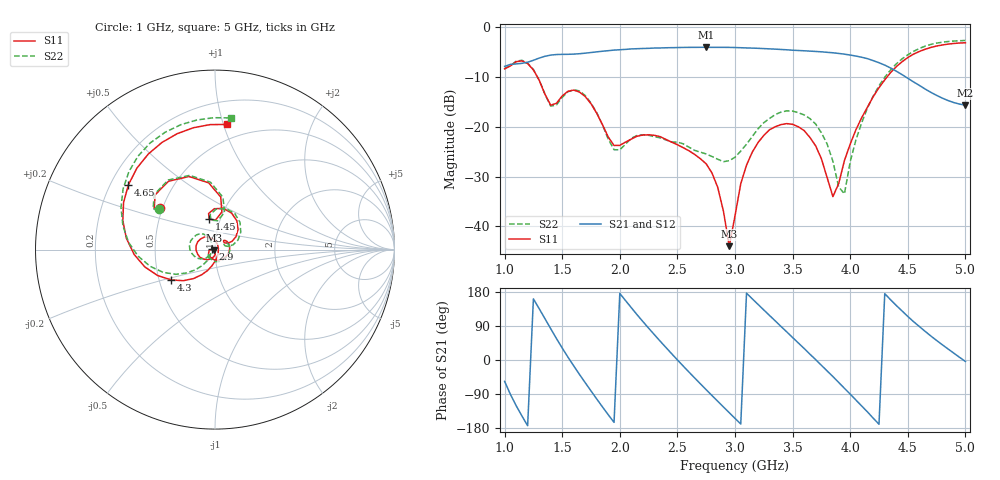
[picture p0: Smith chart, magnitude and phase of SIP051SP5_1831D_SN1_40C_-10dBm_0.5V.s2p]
# GHz  S  dB  R  50
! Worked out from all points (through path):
!   81 points, 1 GHz to 5 GHz, reference 50 ohm
!   highest |S21| = -4.00 dB at 2.75 GHz (marker M1); lowest = -15.6 dB at 5 GHz (marker M2)
!   lowest |S11| = -44.0 dB at 2.95 GHz (marker M3), VSWR 1.01, Z = 49.5 - j0.31 ohm
!   |S11| at or under -10 dB: 1.285 GHz to 4.319 GHz (3.034 GHz wide, 108 % of centre)
!   |S22| runs from -33.5 to -2.6 dB; largest |S21 - S12| = 0.0046
!   S11 on the Smith chart (normalised r, x): 1 GHz: 0.49, +0.26; 1.45 GHz: 0.89, +0.31; 2.9 GHz: 0.97, +0.00; 4.3 GHz: 0.58, -0.21; 4.65 GHz: 0.27, +0.31; 5 GHz: 0.37, +1.02
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1  -8.33 142.8  -7.83 -56.3  -7.83 -56.7  -8.27 143.9
1.25  -8.55 95.4  -6.61 161.3  -6.61 161.5  -8.48 93.9
1.45  -15.28 100.6  -5.46 56.7  -5.45 56.7  -15.60 97.6
1.7  -13.91 52.9  -5.18 -60.0  -5.19 -60.1  -13.71 47.5
1.85  -19.59 25.8  -4.79 -124.0  -4.79 -123.9  -19.67 14.8
2  -23.74 45.4  -4.49 175.7  -4.48 175.7  -24.63 30.8
2.2  -21.65 26.6  -4.24 101.6  -4.25 101.5  -21.61 8.9
2.35  -21.98 -10.2  -4.13 49.8  -4.13 49.8  -22.23 -31.8
2.55  -24.20 -74.2  -4.03 -15.8  -4.04 -15.8  -23.42 -85.7
2.75  -27.45 -148.2  -4.00 -78.4  -4.01 -78.4  -25.46 -133.7
2.9  -37.02 174.5  -4.01 -124.0  -4.02 -123.8  -27.02 -147.5
2.95  -44.02 -150.2  -4.02 -139.0  -4.03 -139.1  -26.82 -144.2
3  -37.92 -87.7  -4.05 -154.0  -4.05 -154.0  -26.12 -138.0
3.15  -25.09 -113.0  -4.16 161.4  -4.16 161.5  -21.95 -141.6
3.35  -19.98 -165.3  -4.37 103.0  -4.39 102.9  -17.53 -172.1
3.7  -23.82 103.4  -4.84 1.1  -4.84 1.0  -19.44 126.4
3.85  -34.05 15.8  -5.10 -43.7  -5.11 -44.0  -26.94 117.2
3.95  -26.79 -75.8  -5.38 -74.7  -5.39 -74.8  -33.48 -156.1
4.3  -10.55 -145.3  -7.58 175.1  -7.59 175.0  -10.02 -156.3
4.35  -9.10 -155.7  -8.17 159.2  -8.17 159.4  -8.57 -165.5
4.65  -4.40 143.2  -12.39 75.7  -12.40 75.7  -3.77 137.7
5  -3.10 84.7  -15.63 -3.8  -15.67 -4.1  -2.62 83.0
